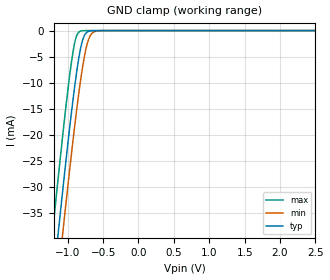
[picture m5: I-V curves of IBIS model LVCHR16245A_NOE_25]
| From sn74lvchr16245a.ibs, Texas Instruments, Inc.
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[Model]   LVCHR16245A_NOE_25
Model_type  Input
Vinl=0.7
Vinh=1.7
| variable   typ   min   max
C_comp   3.45pF   2.65pF   4.59pF
[Temperature Range]   40   100   -40
| Ambient temperature   25   85   -40
[Voltage range]   2.5   2.3   2.7
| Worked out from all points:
|   GND clamp passes 1 mA (typ) near -0.77 V on its own axis
[GND Clamp]
| LVCHR16245A_NOE_25
|   Voltage   I(typ)   I(min)   I(max)
-5.5V     -655.2mA   -662.2mA   -646.6mA
-1.215V   -49.6mA    -57.88mA   -38.96mA
-1.14V    -39.72mA   -48.01mA   -29.07mA
-1.12V    -37.12mA   -45.41mA   -26.48mA
-1.08V    -31.98mA   -40.25mA   -21.38mA
-1.06V    -29.44mA   -37.69mA   -18.89mA
-960mV    -17.26mA   -25.26mA   -7.377mA
-890mV    -9.597mA   -17.1mA    -1.734mA
-785mV    -1.671mA   -6.635mA   -21.67uA
-720mV    -242.5uA   -2.354mA   -1.023uA
-650mV    -22.01uA   -443.9uA   -37.93nA
2.5V      4.713pA    7.577pA    4.389pA
